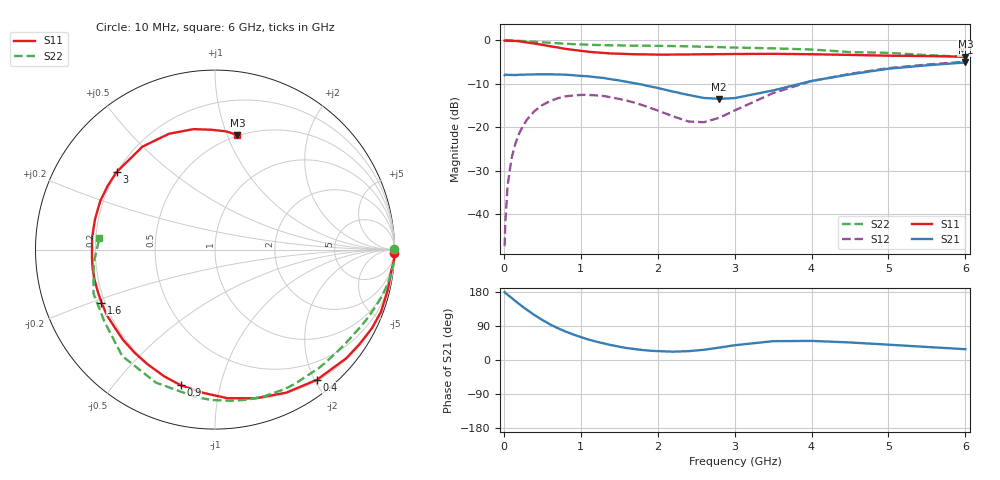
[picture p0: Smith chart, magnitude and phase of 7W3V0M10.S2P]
! Infineon Technologies  Discrete & RF Semiconductors
! BFS17W
! Si NPN RF Bipolar Junction Transistor in SOT323
! VCE = 3 V  IC = 0.1 mA
! Common Emitter S-Parameters:  August  1999
# GHz  S  MA  R  50
!  f  S11  S21  S12  S22
! GHz  MAG  ANG  MAG  ANG  MAG  ANG  MAG  ANG
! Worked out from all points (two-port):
!   36 points, 10 MHz to 6 GHz, reference 50 ohm
!   highest |S21| = -5.07 dB at 6 GHz (marker M1); lowest = -13.4 dB at 2.8 GHz (marker M2)
!   |S21| within 3 dB of the highest: start of sweep to 942.2 MHz; 4.414 GHz to end of sweep
!   lowest |S11| = -3.7 dB at 6 GHz (marker M3), VSWR 4.72, Z = 24.6 + j54.4 ohm
!   |S11| at or under -10 dB: nowhere
!   |S22| runs from -3.8 to 0.0 dB; largest |S21 - S12| = 0.4
!   S11 on the Smith chart (normalised r, x): 10 MHz: 21, -91; 400 MHz: 0.21, -2.03; 900 MHz: 0.20, -0.76; 1.6 GHz: 0.19, -0.21; 3 GHz: 0.20, +0.33; 6 GHz: 0.49, +1.09
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0.01  0.9951 -1.2  0.398 179.2  0.0043 84.6  0.9999 0.1
0.02  0.9999 -3.0  0.405 176.7  0.0083 89.4  0.9952 -0.8
0.05  0.9896 -6.7  0.402 172.0  0.0218 86.5  0.9984 -2.0
0.1  0.9882 -13.2  0.401 164.1  0.0439 81.4  0.9998 -4.0
0.2  0.9779 -26.6  0.403 147.7  0.0855 73.0  0.9894 -7.9
0.3  0.9496 -39.6  0.405 132.5  0.1227 64.3  0.9792 -11.7
0.4  0.921 -52.0  0.407 118.3  0.1547 56.3  0.9666 -15.3
0.6  0.8585 -74.8  0.408 94.1  0.2011 42.9  0.9397 -21.9
0.9  0.7794 -104.2  0.398 67.4  0.2326 26.5  0.9068 -31.0
1.1  0.7409 -120.6  0.387 54.0  0.2364 18.3  0.8933 -36.8
1.3  0.718 -135.5  0.37 43.7  0.2295 11.6  0.8822 -42.9
1.6  0.6984 -155.0  0.334 31.5  0.2029 4.6  0.8724 -51.8
2.2  0.688 174.4  0.258 22.0  0.1339 9.6  0.862 -71.1
2.6  0.6941 157.1  0.218 27.0  0.1147 36.1  0.846 -84.5
2.8  0.6954 149.2  0.213 32.7  0.1288 50.0  0.8384 -91.2
3  0.6982 141.8  0.217 38.9  0.1564 59.2  0.8287 -97.4
3.5  0.7016 125.1  0.266 49.7  0.2481 64.7  0.8108 -114.0
4  0.6943 111.6  0.342 50.4  0.3409 59.3  0.7868 -131.1
4.5  0.6818 100.1  0.407 46.3  0.4132 51.6  0.7352 -146.9
5  0.6679 91.6  0.473 40.4  0.4808 44.1  0.7198 -160.2
5.5  0.6614 84.5  0.518 34.4  0.5277 36.8  0.679 -173.9
6  0.6504 78.9  0.558 28.5  0.5689 30.2  0.6475 174.2
